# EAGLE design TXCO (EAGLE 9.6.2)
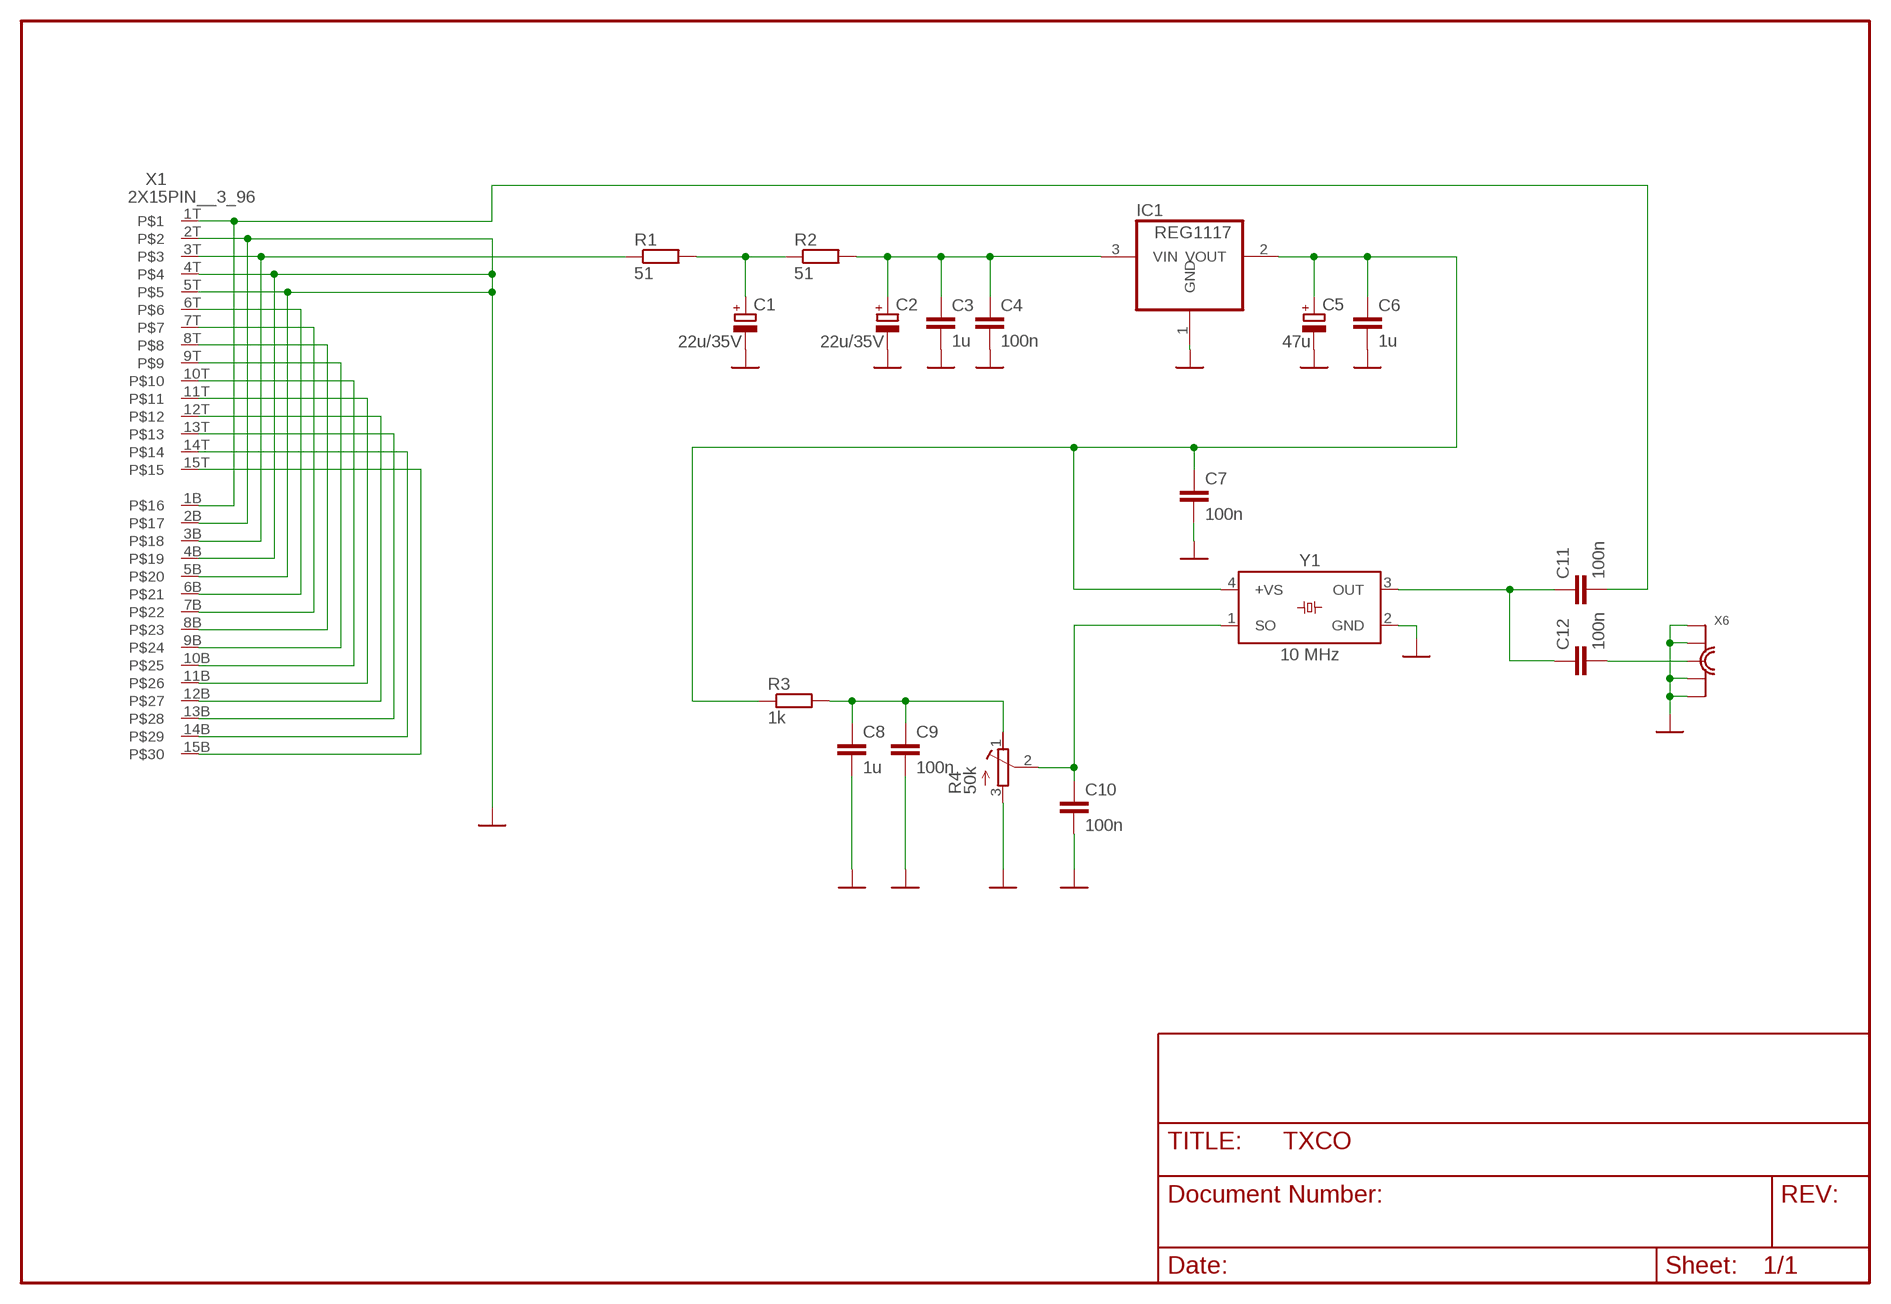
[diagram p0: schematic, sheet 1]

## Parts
C1  22u/35V  CPOL-EUD/7343-31R  [D/7343-31R]
C2  22u/35V  CPOL-EUD/7343-31R  [D/7343-31R]
C3  1u  C-EUC0805K  [C0805K]
C4  100n  C-EUC0805K  [C0805K]
C5  47u  CPOL-EUD/7343-31R  [D/7343-31R]
C6  1u  C-EUC0805K  [C0805K]
C7  100n  C-EUC0805K  [C0805K]
C8  1u  C-EUC0805K  [C0805K]
C9  100n  C-EUC0805K  [C0805K]
C10  100n  C-EUC0805K  [C0805K]
C11  100n  C-EUC0805K  [C0805K]
C12  100n  C-EUC0805K  [C0805K]
IC1  REG1117  [SOT223]
R1  51  R-EU_0207/10  [0207/10]
R2  51  R-EU_0207/10  [0207/10]
R3  1k  R-EU_M0805  [M0805]
R4  50k  R-TRIMM3006P  [RTRIM3006P]
X1  2X15PIN__3_96  [15PIN__3_96__FEMALE]
X6  MMCX_BU_VERT  [MMCX]
Y1  10 MHz  WE-SPXO_CFPS-73_831020184  [WE-SPXO_CFPS-73]

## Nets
GND: C1.- C2.- C3.2 C4.2 C5.- C6.2 C7.2 C8.2 C9.2 C10.2 IC1.1(GND) R4.3(A) X1.2B X1.2T X1.4B X1.4T X1.5B X1.5T X6.GND1 X6.GND2 X6.GND3 X6.GND4 Y1.2(GND)
N$1: C11.2 X1.1B X1.1T
N$2: C8.1 C9.1 R3.2 R4.1(E)
N$3: R1.1 X1.3B X1.3T
N$4: C10.1 R4.2(S) Y1.1(SO)
N$5: C12.2 X6.INNEN
N$6: X1.6B X1.6T
N$7: X1.7B X1.7T
N$8: X1.8B X1.8T
N$9: X1.9B X1.9T
N$10: X1.10B X1.10T
N$11: X1.11B X1.11T
N$12: X1.12B X1.12T
N$13: X1.13B X1.13T
N$14: X1.14B X1.14T
N$15: X1.15B X1.15T
N$16: C1.+ R1.2 R2.1
N$17: C2.+ C3.1 C4.1 IC1.3(VIN) R2.2
N$18: C5.+ C6.1 C7.1 IC1.2(VOUT) R3.1 Y1.4(+VS)
N$19: C11.1 C12.1 Y1.3(OUT)

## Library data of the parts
C1 C2 C5 = rcl:CPOL-EU: POLARIZED CAPACITOR, European symbol; SPICEPREFIX: C
C3 C4 C6-C12 = rcl:C-EU: CAPACITOR, European symbol; SPICEPREFIX: C
IC1 = burr-brown:REG1117: 800mA and 1A Low Dropout (LDO) Positive Regulator 1.8V, 2.5V, 2.85V, 3.3V, 5V, and Adj; MPN: REG1117; OC_FARNELL: 1097566; OC_NEWARK: 14P6981
R1-R3 = rcl:R-EU_: RESISTOR, European symbol; SPICEPREFIX: R
R4 = rcl:R-TRIMM: Trimm resistor; SPICEMODEL: X; SPICEPREFIXL: POT
X1 = jamma:2X15PIN__3_96: 2x 15pin 3.96 PCB edge connector male, HP OCXO
X6 = con-bkm:MMCX_BU_VERT
Y1 = Eagle_WE-SPXO (rev25a):WE-SPXO_CFPS-73: WE-SPXO Simple Packaged Quartz Oscillator Characteristics SMT models Hermetically sealed Frequencies between 3.6864 MHz and 156.25 MHz plus 32.768 kHz Maximum operating temperatures range: -40 °C to 125 °C Stabilities down to ±25 ppm available Available supply voltages: 1.8 V; 2.5 V; 3.3 V; 5 V and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; DATASHEET-URL: https://www.we-online.com/redexpert/spec/831020184?ae; FREQUENCY: 14.31818 MHz; HEIGHT: 1.8mm; LENGTH: 7mm; MOUNT: SMT; OPERATING-TEMPERATURE: -40 °C up to +85 °C; OUTPUT-LOGIC: CMOS; PART-NUMBER: 831020184; SIZE: CFPS-73; STABILITY: 50ppm; V-SUPPLY: 3.3 V; VALUE: 14.31818 MHz; WIDTH: 5mm

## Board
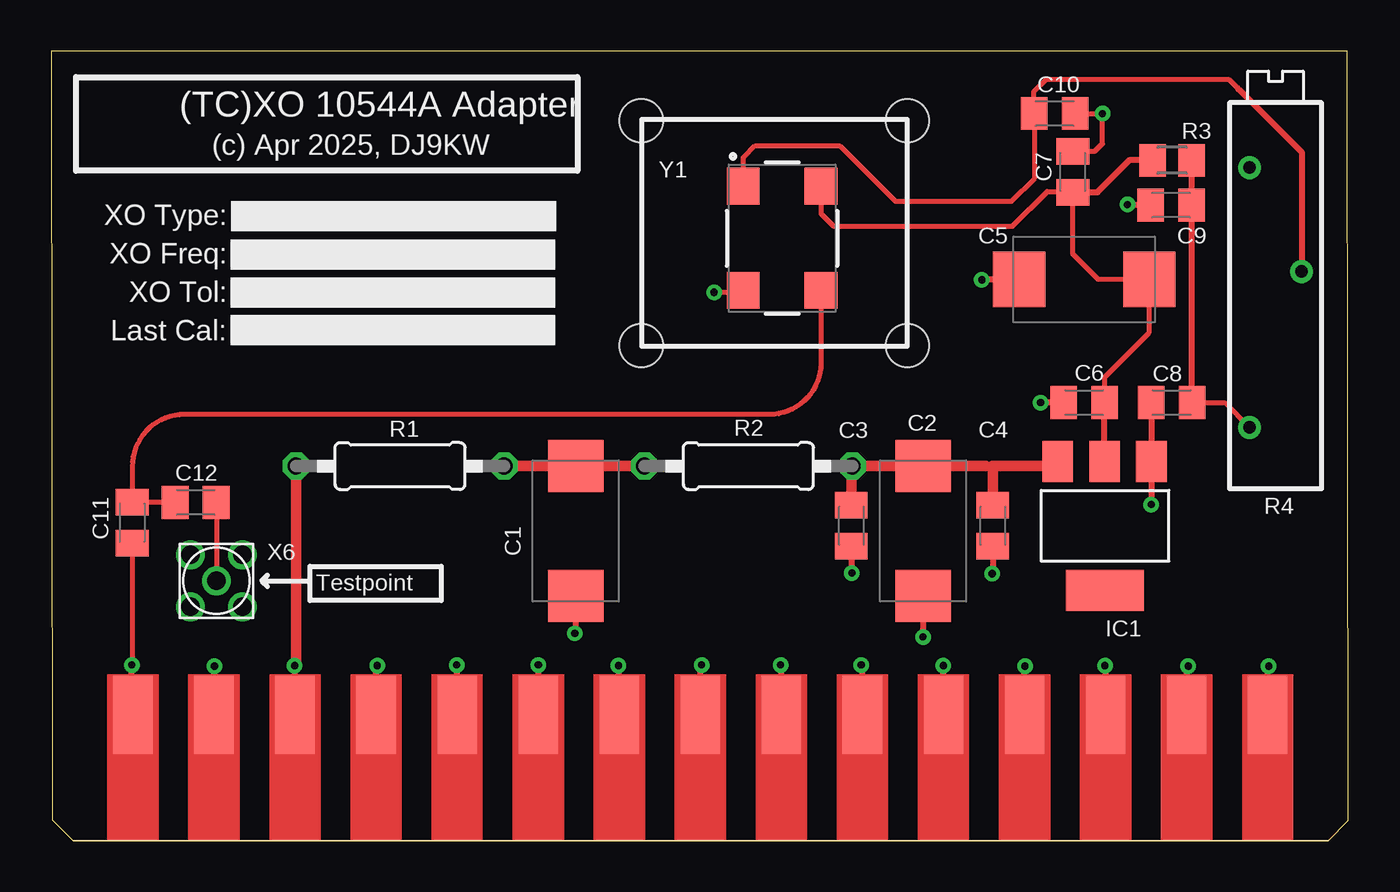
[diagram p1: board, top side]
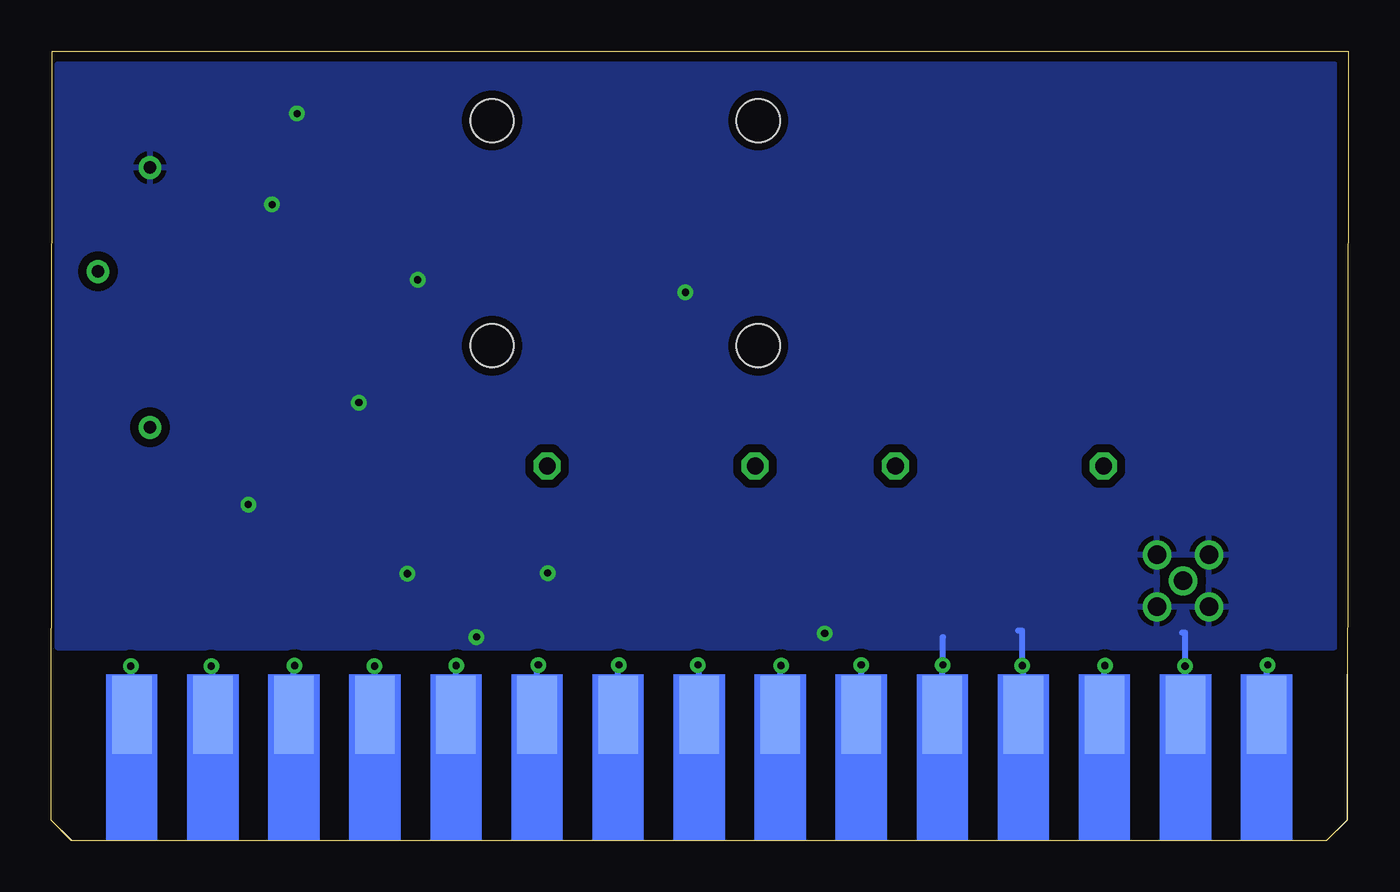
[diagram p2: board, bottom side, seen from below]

Size 63.37 x 38.58 mm. Coordinates in mm from the lower left corner, seen from the top.
Outline: 0.05,1.02 1.07,0 62.38,0 63.37,0.99 63.32,38.58 0,38.58 0.05,1.02
Copper layers (1*16): Top 0.035mm / dielectric 1.5mm / Bottom 0.035mm
Design rules "BM 2lagig *": minimum track width 10mil, minimum drill 0.2mm, track to track 5mil, track to pad 5mil, pad to pad 5mil, via to via 5mil, smd to smd 0mil, copper to edge 0mil, drill to drill 8mil, minimum pad ring 10mil, minimum via ring 8mil, stop-mask expansion 4mil, vias tented up to drill 0mil, thermal gap 10mil
Holes 2.1 mm at 28.83,24.19 41.83,24.19 28.83,35.19 41.83,35.19

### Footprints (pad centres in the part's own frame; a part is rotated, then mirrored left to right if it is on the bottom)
D/7343-31R = smd 2.55 x 2.7: + 3.175,0; - -3.175,0
C0805K = smd 1.3 x 1.6: 1 -1,0; 2 1,0
SOT223 = smd 1.499 x 2.007: 1 -2.261,-3.15; 2 0.025,-3.15; 3 2.311,-3.15 | smd 3.81 x 2.007: 4 0,3.15
0207/10 = drill 0.813 octagon: 1 -5.08,0; 2 5.08,0
M0805 = smd 1.3 x 1.6: 1 -0.95,0; 2 0.95,0
RTRIM3006P = drill 0.61: 1 -7.62,1.27; 2 0,-1.27; 3 5.08,1.27
15PIN__3_96__FEMALE = smd 1.93 x 3.81 bottom: 1B -22.98,-0.71; 2B -19.02,-0.71; 3B -15.06,-0.71; 4B -11.1,-0.71; 5B -7.14,-0.71; 6B -3.18,-0.71; 7B 0.78,-0.71; 8B 4.74,-0.71; 9B 8.7,-0.71; 10B 12.66,-0.71; 11B 16.62,-0.71; 12B 20.58,-0.71; 13B 24.54,-0.71; 14B 28.5,-0.71; 15B 32.46,-0.71 | smd 1.93 x 3.81: 1T -22.98,-0.71; 2T -19.02,-0.71; 3T -15.06,-0.71; 4T -11.1,-0.71; 5T -7.14,-0.71; 6T -3.18,-0.71; 7T 0.78,-0.71; 8T 4.74,-0.71; 9T 8.7,-0.71; 10T 12.66,-0.71; 11T 16.62,-0.71; 12T 20.58,-0.71; 13T 24.54,-0.71; 14T 28.5,-0.71; 15T 32.46,-0.71
MMCX = drill 0.9: GND1 -1.27,1.27; GND2 1.27,1.27; GND3 -1.27,-1.27; GND4 1.27,-1.27; INNEN 0,0
WE-SPXO_CFPS-73 = smd 1.8 x 1.6: 1 -2.54,-1.9; 2 2.54,-1.9; 3 2.54,1.9; 4 -2.54,1.9

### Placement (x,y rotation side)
C1  25.63,15.14 90 top
C2  42.6,15.14 90 top
C3  39.09,15.39 270 top
C4  46,15.39 270 top
C5  50.47,27.43 0 top
C6  50.47,21.41 180 top
C7  49.91,32.69 90 top
C8  54.74,21.41 180 top
C9  54.71,31.06 180 top
C10  49.02,35.53 0 top
C11  3.96,15.54 270 top
C12  7.06,16.54 0 top
IC1  51.49,15.39 180 top
R1  17.04,18.31 0 top
R2  34.06,18.31 0 top
R3  54.76,33.25 0 top
R4  59.82,27.81 90 top
X1  26.97,6.87 0 top
X6  8.08,12.7 0 top
Y1  35.71,29.44 270 top

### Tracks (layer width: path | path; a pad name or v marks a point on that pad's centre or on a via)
GND  (via drill 0.35)
  Top 0.254: C10.2 51.33,35.53 | 51.33,35.53 v51.36,35.53 | C7.2 50.99,33.69 51.36,34.06 51.36,35.51 51.33,35.53 | Y1.2 33.71,26.8 v32.38,26.8
  Top 0.305: v7.98,8.53 7.95,8.51 X1.2T | X1.4B 15.87,8.51 v15.93,8.56 | X1.5T 19.83,8.56 v19.81,8.59 | C1.- 25.63,10.18 v25.58,10.13 | C9.2 52.6,31.06 v52.58,31.09 | v53.75,16.43 IC1.1 53.74,18.55 C8.2 | C6.2 v48.34,21.41 | C5.- 45.49,27.43 v45.47,27.41 | C2.- v42.6,9.95 | C3.2 39.09,13.1 v39.12,13.08 | C4.2 46,13.05 v45.97,13.05
  Bottom 0.305: X1.2T 7.95,8.51 v7.98,8.53 7.98,10.16 8.13,10.16 | X1.4B 15.87,8.51 v15.93,8.56 15.93,10.26 16.13,10.26 | X1.5T 19.83,8.56 v19.81,8.59 19.81,9.96 19.79,9.96
  pour Bottom (isolate 0.406): 0.69,37.92 63.07,37.92 63.07,9.45 0.69,9.45
N$1  (via drill 0.35)
  Top 0.254: C11.2 3.96,8.61 v3.94,8.59
  Top 0.305: X1.1T 3.94,6.22 v3.94,8.59
  Bottom 0.305: X1.1T 3.99,8.53 v3.94,8.59
N$2
  Top 0.254: C8.1 57.33,21.41 R4.1
  Top 0.305: R3.2 C9.1 55.71,21.44 C8.1
N$3  (via drill 0.35)
  Top 0.305: 11.91,8.53 v11.89,8.56 | X1.3T 11.91,8.53 | 11.96,8.58 11.91,8.53
  Top 0.508: R1.1 11.96,8.58
  Bottom 0.305: X1.3T 11.91,8.53 v11.89,8.56
N$4
  Top 0.254: 58.1,36.64 57.53,37.21 48.62,37.21 48.02,36.62 C10.1 48.06,35.5 48.06,32.39 46.91,31.24 41.25,31.24 38.53,33.96 34.39,33.96 33.81,33.38 Y1.1
  Top 0.305: R4.2 61.09,33.66 58.1,36.64 57.96,36.78
N$5
  Top 0.254: C12.2 8.08,16.54 X6.INNEN
N$6  (via drill 0.35)
  Top 0.305: X1.6T v23.8,8.59
  Bottom 0.305: X1.6T v23.79,8.58 v23.8,8.59
N$7  (via drill 0.35)
  Top 0.305: X1.7T 27.75,8.52 v27.71,8.56
  Bottom 0.305: X1.7T 27.75,8.52 v27.71,8.56
N$8  (via drill 0.35)
  Top 0.305: X1.8T 31.71,8.52 v31.78,8.59
  Bottom 0.305: X1.8T 31.71,8.52 v31.78,8.59
N$9  (via drill 0.35)
  Top 0.305: X1.9T 35.67,8.55 v35.64,8.59
  Bottom 0.305: X1.9T 35.67,8.55 v35.64,8.59
N$10  (via drill 0.35)
  Top 0.305: X1.10T 39.63,8.52 v39.57,8.59
  Bottom 0.305: X1.10T 39.63,8.52 v39.57,8.59
N$11  (via drill 0.35)
  Top 0.305: X1.11T 43.59,8.55 v43.59,8.56
  Bottom 0.305: X1.11T 43.59,8.55 v43.59,8.56
N$12  (via drill 0.35)
  Top 0.305: X1.12T 47.55,8.52 v47.57,8.53
  Bottom 0.305: X1.12T 47.55,8.52 v47.57,8.53
N$13  (via drill 0.35)
  Top 0.305: X1.13T 51.51,8.53 v51.49,8.56
  Bottom 0.305: X1.13T 51.51,8.53 v51.49,8.56
N$14  (via drill 0.35)
  Top 0.305: X1.14T 55.47,8.46 v55.55,8.53
  Bottom 0.305: X1.14T 55.47,8.46 v55.55,8.53
N$15  (via drill 0.35)
  Top 0.305: X1.15T 59.43,8.48 v59.49,8.53
  Bottom 0.305: X1.15T 59.43,8.48 v59.49,8.53
N$16
  Top 0.305: 25.17,18.31 C1.+
  Top 0.508: R1.2 25.17,18.31 | R2.1 C1.+
N$17
  Top 0.305: 39.09,18.26 R2.2 | 45.67,18.31 45.97,18.31 46,18.29 | IC1.3 48.95,18.31
  Top 0.508: R2.2 C2.+ 45.67,18.31 | C3.1 39.09,18.26 | 46,18.29 C4.1 | 48.95,18.31 45.97,18.31
N$18
  Top 0.254: C6.1 51.47,22.67 53.64,24.84 C5.+ 51.16,27.43 49.91,28.68 C7.1 49.88,31.72 48.67,31.72 46.96,30.02 38.23,30.02 37.61,30.64 Y1.4 37.9,31.69
  Top 0.305: IC1.2 51.46,21.4 C6.1 | R3.1 53.79,33.27 52.7,33.27 51.12,31.69 C7.1 | C7.1 50.05,31.55 50.44,31.55 | C7.1 50.44,31.16
N$19
  Top 0.254: Y1.3 37.61,23.37 arc-90 35.07,20.83 6.5,20.83 arc90 3.96,18.29 C11.1 C12.1

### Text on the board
tPlace: (TC)XO 10544A Adapter | (c) Apr 2025, DJ9KW | XO Type: | XO Freq: | XO Tol: | Last Cal: | Testpoint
